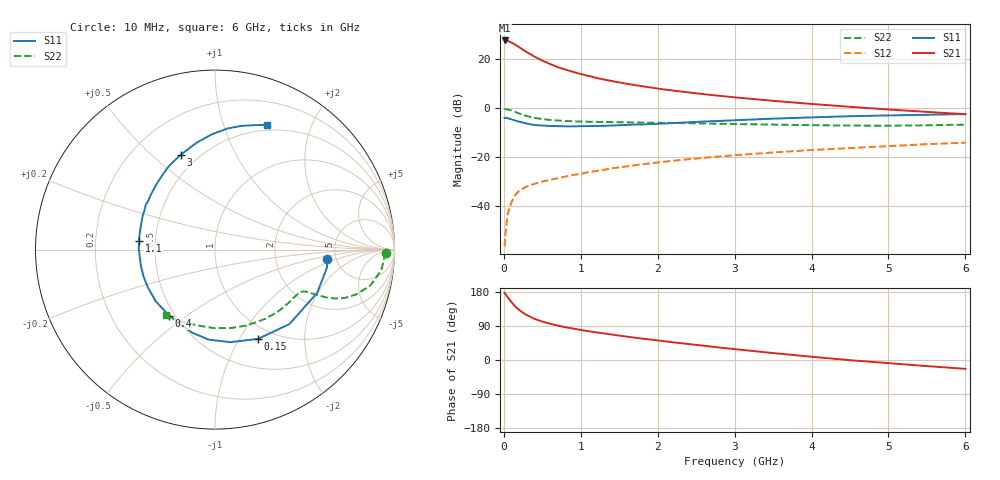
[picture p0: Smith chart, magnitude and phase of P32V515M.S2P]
! SIEMENS Small Signal Semiconductors
! BFP181
! Si NPN RF Bipolar Junction Transistor in SOT143
! VCE = 2.5 V  IC = 15 mA
! Common Emitter S-Parameters:  March  1996
# GHz  S  MA  R  50
!  f  S11  S21  S12  S22
! GHz  MAG  ANG  MAG  ANG  MAG  ANG  MAG  ANG
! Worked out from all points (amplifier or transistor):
!   36 points, 10 MHz to 6 GHz, reference 50 ohm
!   highest |S21| = 27.6 dB at 10 MHz (marker M1)
!   |S21| within 3 dB of that: start of sweep to 211.1 MHz
!   unconditionally stable (mu >= 1): 641.7 MHz to end of sweep
!   at 250 MHz: K = 0.52, MSG = 28.3 dB, |S12| = -32.9 dB
!   at 1.4 GHz: K = 1.31, MAG = 14.5 dB, |S12| = -24.7 dB
!   at 6 GHz: K = 1.07, MAG = 4.2 dB, |S12| = -14.2 dB
!   S11 on the Smith chart (normalised r, x): 10 MHz: 4.22, -0.73; 150 MHz: 0.84, -1.21; 400 MHz: 0.47, -0.43; 1.1 GHz: 0.40, +0.05; 3 GHz: 0.40, +0.62; 6 GHz: 0.44, +1.40
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0.01  0.6267 -4.8  24 177.0  0.0015 86.0  0.9506 -1.1
0.02  0.6318 -9.1  23.97 174.4  0.0026 87.7  0.9444 -2.6
0.05  0.6182 -23.0  23.52 165.5  0.0069 84.2  0.934 -7.0
0.1  0.5865 -45.1  21.64 152.5  0.012 69.4  0.8882 -13.0
0.15  0.5522 -64.2  19.56 141.0  0.0169 63.2  0.8276 -17.5
0.2  0.523 -80.5  17.46 131.9  0.0203 58.6  0.7723 -20.4
0.25  0.5027 -94.1  15.42 124.3  0.0227 55.6  0.7235 -22.1
0.3  0.4793 -105.8  13.77 118.4  0.025 53.0  0.6845 -23.1
0.4  0.4486 -124.6  11.18 108.5  0.0283 50.9  0.6287 -23.9
0.5  0.4381 -139.0  9.271 101.4  0.0313 49.9  0.5932 -24.3
0.6  0.4294 -150.8  7.942 95.7  0.034 50.3  0.5702 -24.6
0.7  0.4253 -159.8  6.844 90.8  0.0368 51.6  0.5547 -24.9
0.9  0.4212 -174.7  5.475 83.0  0.0428 52.7  0.5349 -26.1
1.1  0.4267 173.5  4.523 76.0  0.0489 53.5  0.524 -27.9
1.3  0.4321 163.9  3.818 70.1  0.0547 53.4  0.5168 -30.2
1.5  0.4446 155.2  3.329 64.3  0.0612 53.7  0.5114 -32.5
2.2  0.4913 131.0  2.27 46.7  0.0835 51.3  0.494 -43.1
3  0.5617 109.9  1.652 28.7  0.1082 46.3  0.4698 -57.3
3.5  0.6052 99.6  1.4 18.3  0.1233 42.9  0.4576 -67.6
4.5  0.6789 84.0  1.057 -0.5  0.1518 34.9  0.4373 -90.8
5.5  0.726 72.7  0.832 -16.1  0.1821 27.4  0.4429 -115.0
6  0.7522 67.5  0.747 -23.3  0.196 22.8  0.4571 -127.0
